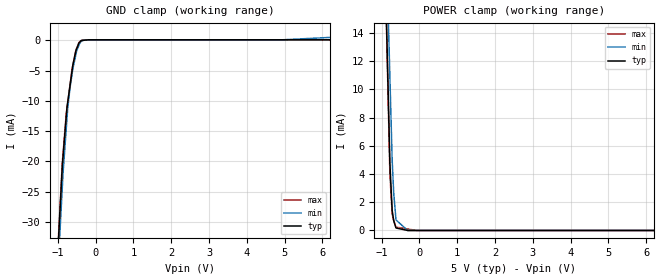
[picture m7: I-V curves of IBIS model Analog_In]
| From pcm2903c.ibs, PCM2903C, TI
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[Model] Analog_In
Model_type Input
Vinl  = 200.000mV
Vinh  = 1.20000V
C_comp  2.00000pF 2.00000pF 2.00000pF
| variable   typ   min   max
[Voltage Range]   5.00000V  4.50000V  5.50000V
[POWER Clamp Reference]  5.00000V  4.50000V  5.50000V
[GND Clamp Reference]   0.00000V  0.00000V  0.00000V
[Temperature Range]   25   85   -25
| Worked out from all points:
|   GND clamp passes 1 mA (typ) near -0.48 V on its own axis
|   POWER clamp passes 1 mA (typ) near -0.70 V on its own axis
[GND Clamp]
-5V       -516.7mA   -511.3mA   -516.9mA
-881.1mV  -20.69mA   -24.2mA    -20.2mA
-861mV    -19.12mA   -21.83mA   -18.62mA
-780.2mV  -12.77mA   -14.83mA   -12.28mA
-760.1mV  -11.19mA   -13.08mA   -11.31mA
-739.6mV  -10.26mA   -11.31mA   -10.32mA
-679mV    -7.53mA    -7.887mA   -7.391mA
-623.5mV  -5.02mA    -5.556mA   -4.707mA
-522mV    -1.726mA   -2.33mA    -1.604mA
-380.7mV  -26.86uA   -130.3uA   -17.92uA
4.936V    100.6uA    99.12uA    98.92uA
10V       100.6uA    1.685mA    98.92uA
[POWER Clamp]
-5V       474.9mA    423mA      493.3mA
-1.139V   44.73mA    45.92mA    45.58mA
-780.6mV  4.768mA    10.9mA     4.029mA
-719.7mV  1.418mA    4.948mA    1.152mA
-679.5mV  698.8uA    2.661mA    700.7uA
-618.7mV  176.3uA    747.4uA    239uA
-309.4mV  0A         0A         104.4uA
-38.05mV  0A         0A         0A
10V       0A         0A         0A
